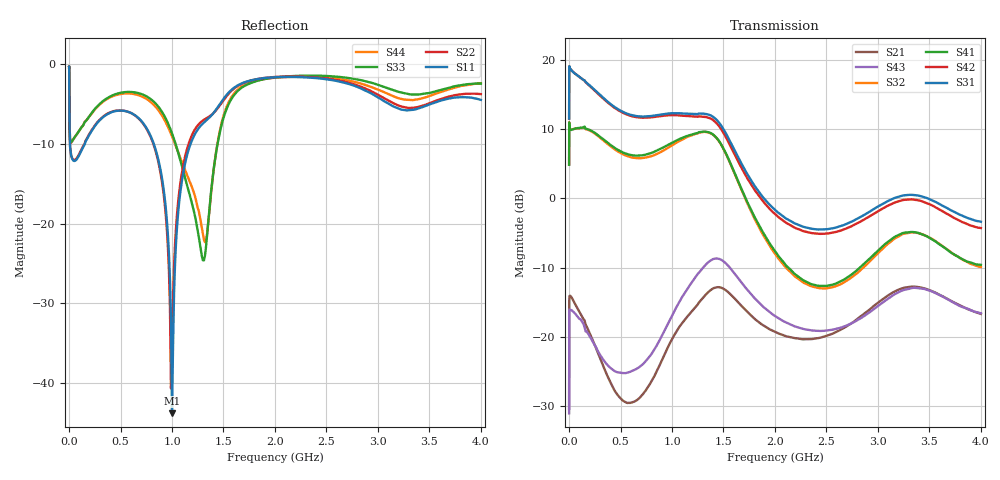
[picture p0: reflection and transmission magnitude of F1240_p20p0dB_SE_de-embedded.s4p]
! Integrated Device Technology
! Corporate Headquarters
! 6024 Silver Creek Valley Road
! San Jose, CA 95138  USA
! Phone:  1-408-284-8200
! Toll Free:  1-800-223-1366
! Webpage:  http://www.idt.com/
! Timing and RF Division
! 515 Groton Road, Suite 102
! Westford, MA 01886-6024
! Device:  F1240
! Description: Dual Intermediate Frequency Digital Variable Gain Amplifier
! Frequency:  10.0 -  500.00 MHz
! Package:  5x5 mm QFN Plastic Package: 32 pin
! Ports:  8 RF, 20 DC
!  Pin  1  = GA3 / Data  Pin 17  = RF OUT_B+
!  Pin  2  = GA4 / CLK  Pin 18  = RF OUT_B-
!  Pin  3  = GA5  Pin 19  = STBY_B
!  Pin  4  = VMODE  Pin 20  = Ground
!  Pin  5  = No Connect  Pin 21  = Ground
!  Pin  6  = GB5  Pin 22  = STB_A
!  Pin  7  = GB4  Pin 23  = RF OUT_A-  = Port 4
!  Pin  8  = GB3  Pin 24  = RF OUT_A+  = Port 3
!  Pin  9  = GB2  Pin 25  = GA0
!  Pin 10  = GB1  Pin 26  = ISET_A
!  Pin 11  = RF IN_B+  Pin 27  = VCC
!  Pin 12  = RF IN_B-  Pin 28  = Ground
!  Pin 13  = Ground  Pin 29  = RF IN_A-  = Port 2
!  Pin 14  = VCC  Pin 30  = RF IN_A+  = Port 1
!  Pin 15  = ISET_B  Pin 31  = GA1
!  Pin 16  = GB0  Pin 32  = GA2 / CSb
! Gain  = +19.5 dB
! State  = 1
! Voltage  = +5.00 V
! Current  = 85.292 mA (one channel only)
! Temperture  =  +25 C
! Test Date  =  2017-10-18
! Board  =  EB4031
! Data:  The device was measured on a custom evaluation board which has
!  individual transmission lines to the RF pins.  Data was collected
!  using a calibrated network analyzer.  The evaluation board was
!  de-embedded using Automatic Fixture Removal.
!  The reference plane is the edge of the package pin.
!  Only Channel A was measured.
!  This data is in single-ended operation.  If your needs are balanced
!  or differential S-parameters then this file needs to be used a
!  linear simulator.
! File Date:  2017-11-10  MJV
! Note:
!  Integrated Device Technology supplies this data as a sample of measured
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# Hz S dB R 100
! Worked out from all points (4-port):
!   410 points, 500 kHz to 4 GHz, reference 100 ohm
!   strongest paths, dB at 500 kHz, 930 MHz, 1.96 GHz, 2.98 GHz, 4 GHz:
!     S31: 11.5, 12.2, -1.1, -1.3, -3.4
!     S42: 11.5, 12.0, -1.7, -2.1, -4.3
!     S41: 4.9, 7.5, -6.8, -7.8, -9.6
!     S32: 4.9, 7.0, -7.1, -8.2, -9.9
!     S43: -31.1, -19.0, -16.6, -15.8, -16.6
!     S21: -30.5, -22.5, -19.0, -15.3, -16.7
!   lowest |S11| = -43.8 dB at 1 GHz (marker M1), VSWR 1.01, Z = 98.8 + j0.461 ohm
!   |S11| at or under -10 dB: 9.214 MHz to 152.3 MHz (143.1 MHz wide, 177 % of centre); 823.5 MHz to 1.18 GHz (356.2 MHz wide, 35.6 % of centre)
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500000  -0.30 -7.0  -30.26 36.1  -27.78 67.3  -63.64 70.9
        -30.46 36.3  -0.29 -6.9  -64.35 65.4  -27.80 68.5
        11.54 -105.7  4.88 72.5  -0.43 0.4  -31.13 178.2
        4.87 73.6  11.52 -104.5  -31.08 178.0  -0.44 2.8
4000000  -7.08 -41.6  -14.18 13.3  -22.80 4.1  -40.06 34.5
         -14.21 13.2  -7.05 -41.7  -40.04 34.3  -22.81 4.1
         18.99 -171.0  10.10 3.0  -6.67 -35.2  -16.09 21.4
         10.08 2.9  18.98 -170.8  -16.08 21.3  -6.73 -35.1
2.1e8  -8.55 -106.0  -19.79 -118.2  -25.51 -51.0  -32.93 10.1
       -19.80 -116.9  -8.45 -107.9  -32.96 10.3  -25.51 -50.9
       16.23 105.6  9.75 -64.1  -6.27 -78.4  -19.58 -128.9
       9.84 -64.0  16.16 104.8  -20.19 -128.3  -6.31 -77.8
5.6e8  -5.91 -170.8  -28.98 88.4  -26.84 -103.1  -27.28 -60.9
       -29.56 86.5  -5.90 -172.1  -27.47 -59.9  -27.02 -103.4
       12.28 19.1  6.16 -149.5  -3.47 -151.0  -24.37 88.1
       6.44 -150.4  12.14 17.9  -25.22 67.6  -3.65 -150.4
1e9  -43.78 158.9  -18.71 -29.8  -23.13 165.4  -22.17 -164.7
     -20.37 -28.9  -38.33 -73.3  -22.55 -160.7  -23.58 164.9
     12.33 -85.7  7.67 116.7  -8.66 145.8  -15.35 -8.4
     8.06 111.5  12.05 -87.6  -16.94 -29.8  -9.02 152.9
1.49e9  -4.51 -132.7  -13.06 165.5  -31.15 52.9  -23.37 68.1
        -12.99 170.9  -4.68 -134.4  -23.48 74.2  -33.68 45.0
        10.24 116.0  7.43 -60.9  -7.16 -100.6  -8.44 167.1
        7.48 -66.2  9.72 114.5  -8.99 159.5  -6.92 -104.1
4e9  -4.46 -159.7  -16.73 51.2  -21.99 -31.2  -19.14 -48.3
     -16.70 50.6  -3.74 -152.6  -21.82 -29.3  -25.67 -9.7
     -3.37 -7.3  -9.93 -153.6  -2.42 -135.7  -14.33 88.6
     -9.61 -163.5  -4.29 1.3  -16.61 62.3  -2.37 -140.1
